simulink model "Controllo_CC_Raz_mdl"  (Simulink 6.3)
settings: Solver=ode45  StartTime=0.0  StopTime=10.0  RelTol=1e-3
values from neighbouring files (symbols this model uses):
  alfa = 0.5+tw1/(2*tan(omega*T/2))    [alfa_beta.m]
  b = k*(T-2*tau1)    (= -1.462)    [Formule_di_Inversione_discrete.m]    (also in Esempio0.m = 0.1; Controllo_CC_K.m = 0.008; motore_CC_ES1.m = 0.8)
  beta = 0.5+tw2/(2*tan(omega*T/2))    [alfa_beta.m]
  Imax = 10000*Amp    (= 10000)    [Controllo_CC_K.m]    (also in motore_CC_ES1.m = 5)
  J = 0.030*kg*m^2    (= 0.03)    [Controllo_CC_K.m]    (also in motore_CC_ES1.m = 1.6)
  K = (1/Ep-1)/G0    [Controllo_CC_K.m]
  Ke = 0.5*N*m/Amp    (= 0.5)    [Controllo_CC_K.m]    (also in motore_CC_ES1.m = 8)
  L = 0.01*Henry    (= 0.01)    [Controllo_CC_K.m]    (also in motore_CC_ES1.m = 0.1)
  R = 1*Ohm    (= 1)    [Controllo_CC_K.m]    (also in motore_CC_ES1.m = 8)
  T = 0.15    [Formule_di_Inversione_discrete.m]    (also in motore_CC_ES1.m = 0.05)
  Tau_r = 0*N*m    (= 0)    [Controllo_CC_K.m]
  Tc = Tfin/2000    (= 2.5e-05)    [Controllo_CC_K.m]
  Vmax = 10000*V    (= 10000)    [Controllo_CC_K.m]    (also in motore_CC_ES1.m = 64)
  Wref = 500*rpm    (= 52.3598775598)    [Controllo_CC_K.m]

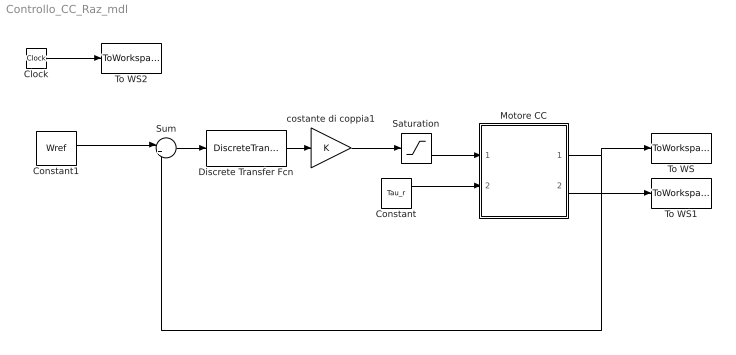
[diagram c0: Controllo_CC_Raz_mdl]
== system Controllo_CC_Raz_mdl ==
  Clock : Clock
  Constant : Constant  Value=Tau_r
  Constant1 : Constant  Value=Wref
  Discrete Transfer Fcn : DiscreteTransferFcn  Numerator=[alfa 1-alfa]  Denominator=[beta 1-beta]  SampleTime=T
  Motore CC : Subsystem
  Saturation : Saturate  UpperLimit=Vmax  LowerLimit=-Vmax
  Sum : Sum  Inputs=|+-
  To WS : ToWorkspace  VariableName=Wm  SampleTime=Tc  SaveFormat=Array
  To WS1 : ToWorkspace  VariableName=Ia  SampleTime=Tc  SaveFormat=Array
  To WS2 : ToWorkspace  VariableName=t  SampleTime=Tc  SaveFormat=Array
  costante di coppia1 : Gain  Gain=K
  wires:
  Constant/1 -> Motore CC/2(Tau_r)
  Clock/1 -> To WS2/1
  Motore CC/1(Wm) -> To WS/1, Sum/2
  Motore CC/2(Ia) -> To WS1/1
  Constant1/1 -> Sum/1
  Sum/1 -> Discrete Transfer Fcn/1
  costante di coppia1/1 -> Saturation/1
  Saturation/1 -> Motore CC/1(Va)
  Discrete Transfer Fcn/1 -> costante di coppia1/1

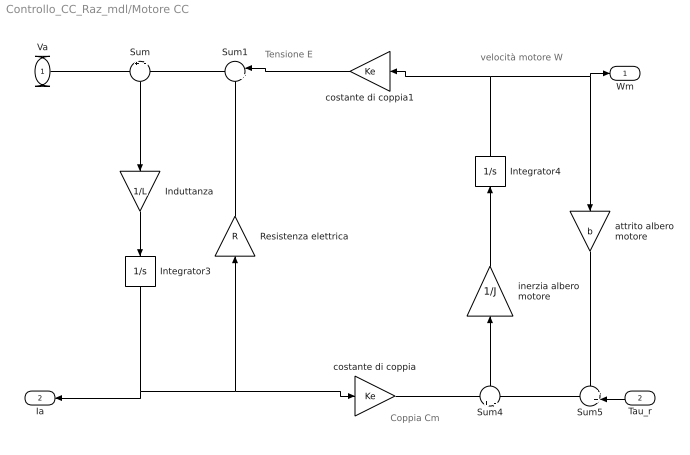
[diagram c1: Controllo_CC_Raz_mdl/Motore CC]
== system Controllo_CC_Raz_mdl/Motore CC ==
  note: Tensione E
  note: velocità motore W
  note: Coppia Cm
  Va : Inport
  Tau_r : Inport  Orientation=left  Port=2
  Induttanza : Gain  Orientation=down  Gain=1/L
  Integrator3 : Integrator  Orientation=down  LimitOutput=on  UpperSaturationLimit=Imax  LowerSaturationLimit=-Imax
  Integrator4 : Integrator  Orientation=up
  Resistenza elettrica : Gain  Orientation=up  Gain=R
  Sum : Sum  Orientation=down  Inputs=+|-
  Sum1 : Sum  Orientation=left  Inputs=|++
  Sum4 : Sum  Orientation=up  Inputs=+|-
  Sum5 : Sum  Orientation=left  Inputs=++|
  attrito albero motore : Gain  Orientation=down  Gain=b
  costante di coppia : Gain  Gain=Ke
  costante di coppia1 : Gain  Orientation=left  Gain=Ke
  inerzia albero motore : Gain  Orientation=up  Gain=1/J
  Wm : Outport
  Ia : Outport  Orientation=left  Port=2
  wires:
  Sum/1 -> Induttanza/1
  Induttanza/1 -> Integrator3/1
  Sum1/1 -> Sum/2
  Resistenza elettrica/1 -> Sum1/2
  Sum4/1 -> inerzia albero motore/1
  inerzia albero motore/1 -> Integrator4/1
  Sum5/1 -> Sum4/2
  attrito albero motore/1 -> Sum5/1
  Integrator4/1 -> costante di coppia1/1, attrito albero motore/1, Wm/1
  costante di coppia1/1 -> Sum1/1
  costante di coppia/1 -> Sum4/1
  Integrator3/1 -> Resistenza elettrica/1, costante di coppia/1, Ia/1
  Va/1 -> Sum/1
  Tau_r/1 -> Sum5/2
